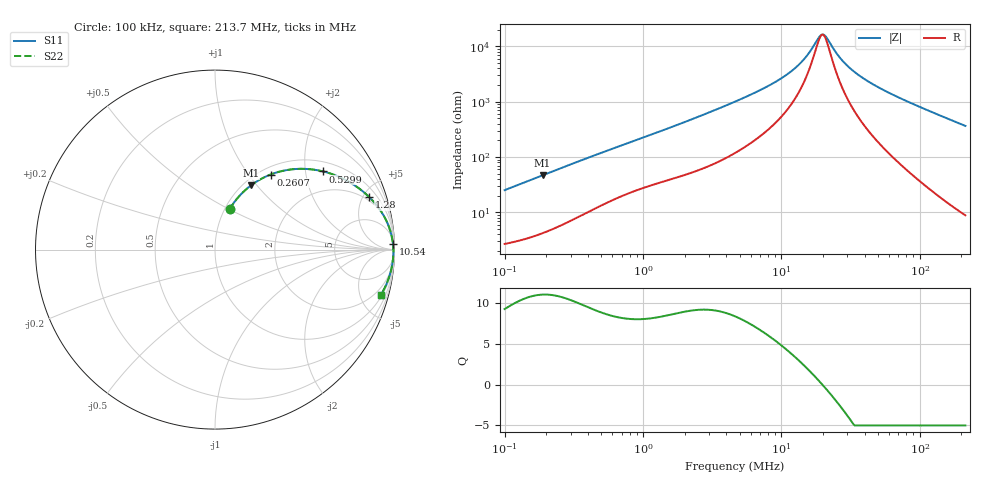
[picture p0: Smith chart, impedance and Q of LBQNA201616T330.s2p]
! LBQNA201616T330  S-PARAMETER MODEL  ( General Type )
! Model Generated by TAIYO YUDEN Corporation (http://www.ty-top.com)
! Version 1.0
! TAIYO YUDEN Control No. 191025NI43SB-FBB
! Copyright(c) 2019 TAIYO YUDEN CO.,LTD. All Rights Reserved.
! Product Description (link to TY-COMPAS)
! https://ds.yuden.co.jp/TYCOMPAS/or/detail?pn=LBQNA201616T330K&u=M
! Products Name : Inductors
! Characteristics :
!  Inductance : 33 uH , SRF(min) : 14 MHz , DC Resistance(max) : 2.21 Ohm
!  Rated Current : Saturation :130 mA , Temp Rise : 140 mA (20 degC)
!  Case Size : 2.0 x 1.6 / 0.079 x 0.063 [mm/inch] , Thickness : 1.6 / 0.063 [mm/inch]
!  (Conditions: Temperature = 25 degC , DC Bias Current/Voltage = 0A / 0V)
! External Node Assignments :
!  1  o---GGG---o  2
! GND o---------o GND
! Frequency Range : 0.1MHz  -  213.673535MHz  [ 402 STEP ]
# MHz S RI R 50
! Freq[MHz].  S11 Real  S11 Imag  S21 Real  S21 Imag  S12 Real  S12 Imag  S22 Real  S22 Imag
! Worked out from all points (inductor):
!   401 points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, 100 kHz to 213.7 MHz, reference 50 ohm
!   read as one part in series: L = 39.8 uH near 103.9 kHz
!   highest Q = 11.1 at 188.2 kHz (marker M1), where L = 39.5 uH
!   self-resonance near 19.46 MHz
!   S11 on the Smith chart (normalised r, x): 100 kHz: 1.05, +0.50; 260.7 kHz: 1.12, +1.28; 529.9 kHz: 1.29, +2.50; 1.28 MHz: 1.67, +5.58; 10.54 MHz: 13, +56; 213.7 MHz: 1.18, -7.29
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0.1  0.0812 0.2247  0.9188 -0.2247  0.9188 -0.2247  0.0812 0.2247
0.188237  0.2012 0.3583  0.7988 -0.3583  0.7988 -0.3583  0.2012 0.3583
0.260747  0.3094 0.4181  0.6906 -0.4181  0.6906 -0.4181  0.3094 0.4181
0.361188  0.4423 0.4485  0.5577 -0.4485  0.5577 -0.4485  0.4423 0.4485
0.529933  0.6019 0.4356  0.3981 -0.4356  0.3981 -0.4356  0.6019 0.4356
0.823534  0.7537 0.3733  0.2463 -0.3733  0.2463 -0.3733  0.7537 0.3733
1.2798  0.8603 0.2915  0.1397 -0.2915  0.1397 -0.2915  0.8603 0.2915
1.304567  0.864 0.2879  0.136 -0.2879  0.136 -0.2879  0.864 0.2879
2.31845  0.942 0.1854  0.058 -0.1854  0.058 -0.1854  0.942 0.1854
4.71194  0.9794 0.0941  0.0206 -0.0941  0.0206 -0.0941  0.9794 0.0941
7.464226  0.9881 0.0555  0.0119 -0.0555  0.0119 -0.0555  0.9881 0.0555
10.53959  0.9914 0.0333  0.00855 -0.0333  0.00855 -0.0333  0.9914 0.0333
13.78367  0.9929 0.0185  0.00707 -0.0185  0.00707 -0.0185  0.9929 0.0185
16.69585  0.9936 0.00863  0.00642 -0.00863  0.00642 -0.00863  0.9936 0.00863
18.73074  0.9938 0.00283  0.00617 -0.00283  0.00617 -0.00283  0.9938 0.00283
20.22332  0.9939 -0.00102  0.00606 0.00102  0.00606 0.00102  0.9939 -0.00102
21.4203  0.994 -0.00392  0.00601 0.00392  0.00601 0.00392  0.994 -0.00392
26.44805  0.994 -0.0148  0.00601 0.0148  0.00601 0.0148  0.994 -0.0148
31.42773  0.9937 -0.0241  0.00626 0.0241  0.00626 0.0241  0.9937 -0.0241
41.10118  0.9928 -0.0402  0.00719 0.0402  0.00719 0.0402  0.9928 -0.0402
60.30341  0.9897 -0.0684  0.0103 0.0684  0.0103 0.0684  0.9897 -0.0684
213.6735  0.9248 -0.2518  0.0752 0.2518  0.0752 0.2518  0.9248 -0.2518
